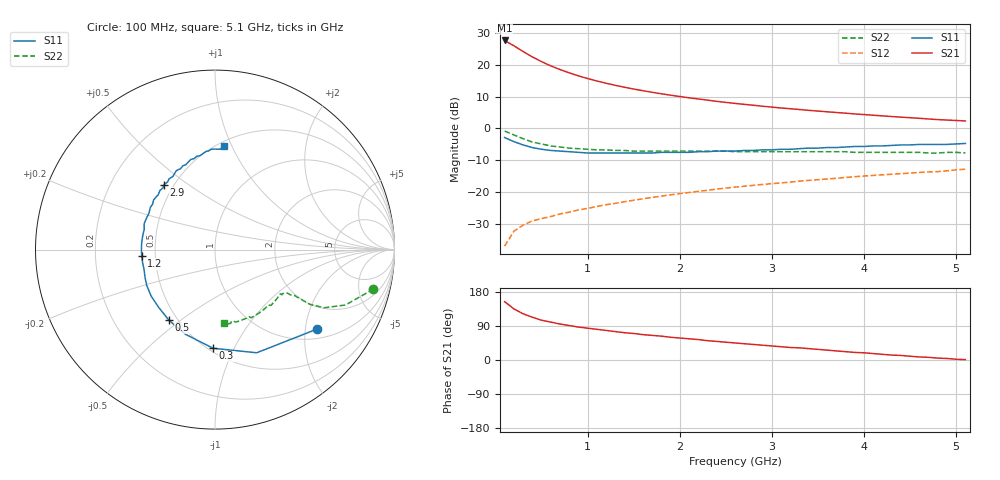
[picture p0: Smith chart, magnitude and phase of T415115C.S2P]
!S-PARAMETERS at Vce=5V  Ic=10mA.  LAST UPDATED 01-25-95
# ghz s ma r 50
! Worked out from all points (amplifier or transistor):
!   51 points, 100 MHz to 5.1 GHz, reference 50 ohm
!   highest |S21| = 27.7 dB at 100 MHz (marker M1)
!   |S21| within 3 dB of that: start of sweep to 273.6 MHz
!   unconditionally stable (mu >= 1): 1.219 GHz to 3.578 GHz
!   at 900 MHz: K = 0.90, MSG = 21.1 dB, |S12| = -25.7 dB
!   at 2.6 GHz: K = 1.08, MAG = 11.5 dB, |S12| = -18.5 dB
!   at 5.1 GHz: K = 0.89, MSG = 7.6 dB, |S12| = -12.8 dB
!   lowest NFmin = 1.10 dB at 100 MHz
!   S11 on the Smith chart (normalised r, x): 100 MHz: 1.26, -2.31; 300 MHz: 0.53, -0.83; 500 MHz: 0.45, -0.45; 1.2 GHz: 0.42, -0.04; 2.9 GHz: 0.44, +0.41; 5.1 GHz: 0.54, +0.94
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0.1  0.72 -38.0  24.27 154.0  0.014 72.0  0.91 -14.0
0.2  0.62 -68.0  20.04 135.0  0.024 62.0  0.79 -23.0
0.3  0.55 -91.0  16.26 122.0  0.03 56.0  0.69 -28.0
0.4  0.5 -109.0  13.39 113.0  0.035 54.0  0.61 -30.0
0.5  0.47 -123.0  11.28 105.0  0.038 53.0  0.57 -30.0
0.6  0.45 -134.0  9.658 100.0  0.041 53.0  0.53 -30.0
0.7  0.44 -144.0  8.473 95.0  0.045 53.0  0.51 -30.0
0.8  0.43 -152.0  7.512 91.0  0.048 54.0  0.49 -31.0
0.9  0.42 -158.0  6.741 87.0  0.052 55.0  0.48 -31.0
1  0.41 -165.0  6.11 84.0  0.055 56.0  0.47 -31.0
1.1  0.41 -170.0  5.587 81.0  0.059 56.0  0.46 -32.0
1.2  0.41 -175.0  5.156 78.0  0.063 57.0  0.46 -32.0
1.4  0.41 176.0  4.45 72.0  0.07 57.0  0.45 -34.0
1.6  0.41 168.0  3.929 67.0  0.078 58.0  0.44 -35.0
1.8  0.42 160.0  3.514 63.0  0.086 58.0  0.44 -37.0
1.9  0.42 157.0  3.338 60.0  0.09 57.0  0.44 -38.0
2.3  0.43 144.0  2.79 51.0  0.106 57.0  0.44 -42.0
2.6  0.44 136.0  2.478 45.0  0.119 56.0  0.43 -46.0
2.9  0.46 128.0  2.237 39.0  0.131 54.0  0.43 -50.0
3.5  0.49 113.0  1.876 28.0  0.156 51.0  0.43 -57.0
4.3  0.54 97.0  1.54 13.0  0.19 46.0  0.42 -69.0
5.1  0.58 85.0  1.31 1.0  0.228 41.0  0.41 -83.0
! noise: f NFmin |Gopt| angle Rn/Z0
0.1  1.1  0.35  10  0.22
0.9  1.3  0.28  68  0.17
1.8  1.6  0.25  149  0.12
2.4  1.8  0.35  -172  0.11
